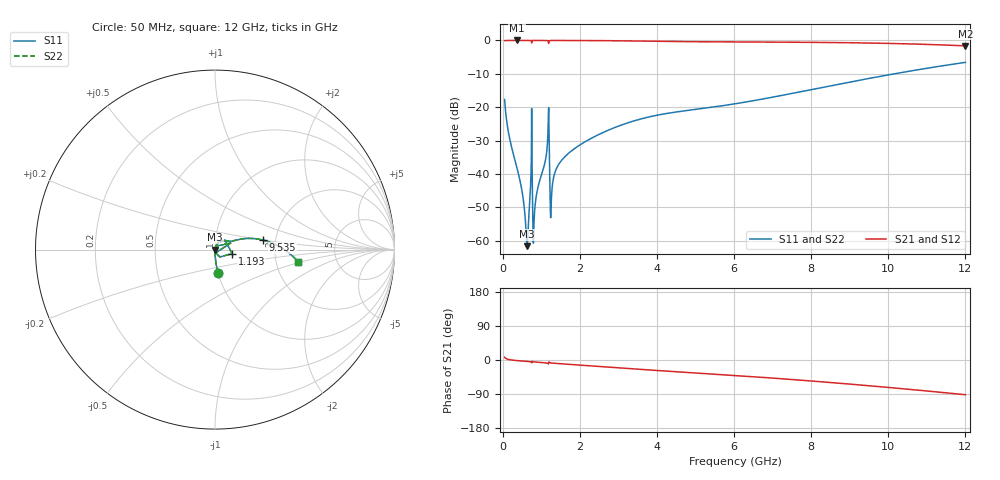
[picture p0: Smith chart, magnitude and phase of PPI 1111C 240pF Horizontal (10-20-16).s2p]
# MHz S MA R 50
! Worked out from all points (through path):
!   1601 points, 50 MHz to 12 GHz, reference 50 ohm
!   highest |S21| = -0.01 dB at 371.2 MHz (marker M1); lowest = -1.6 dB at 12 GHz (marker M2)
!   group delay of S21, straight-line fit = 20.7 ps
!   lowest |S11| = -61.7 dB at 632.6 MHz (marker M3), VSWR 1.00, Z = 50.1 - j0.0101 ohm
!   |S11| at or under -10 dB: start of sweep to 10.16 GHz
!   |S22| runs from -61.7 to -6.6 dB; largest |S21 - S12| = 0
!   S11 on the Smith chart (normalised r, x): 50 MHz: 1.00, -0.26; 1.193 GHz: 1.21, -0.06; 9.535 GHz: 1.71, +0.20; 12 GHz: 2.67, -0.47
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50  0.1303 -82.7  0.9912 7.2  0.9912 7.2  0.1303 -82.7
184.4375  0.03309 -88.4  0.999 0.8  0.999 0.8  0.03309 -88.4
371.1562  0.01226 -88.6  0.9993 -1.5  0.9993 -1.5  0.01226 -88.6
632.5625  0.0008261 -7.0  0.9991 -3.8  0.9991 -3.8  0.0008261 -7.0
669.9062  0.001914 58.4  0.9991 -4.1  0.9991 -4.1  0.001914 58.4
714.7188  0.005271 73.5  0.9989 -4.6  0.9989 -4.6  0.005271 73.5
796.875  0.000917 16.4  0.9991 -4.8  0.9991 -4.8  0.000917 16.4
834.2188  0.003074 68.3  0.9991 -5.2  0.9991 -5.2  0.003074 68.3
908.9062  0.00609 75.2  0.999 -5.8  0.999 -5.8  0.00609 75.2
1095.625  0.01474 76.9  0.9984 -7.4  0.9984 -7.4  0.01474 76.9
1140.438  0.02106 75.3  0.9973 -8.0  0.9973 -8.0  0.02106 75.3
1192.719  0.09836 -13.3  0.9022 -6.5  0.9022 -6.5  0.09836 -13.3
1282.344  0.006215 68.3  0.9984 -8.0  0.9984 -8.0  0.006215 68.3
1357.031  0.01062 74.0  0.9985 -8.7  0.9985 -8.7  0.01062 74.0
1469.062  0.01437 74.6  0.9984 -9.6  0.9984 -9.6  0.01437 74.6
2044.156  0.02812 70.3  0.9966 -13.8  0.9966 -13.8  0.02812 70.3
4038.312  0.07645 41.0  0.9696 -27.9  0.9696 -27.9  0.07645 41.0
6025  0.1124 25.8  0.9496 -40.8  0.9496 -40.8  0.1124 25.8
8019.156  0.1839 19.6  0.9365 -55.5  0.9365 -55.5  0.1839 19.6
9535.312  0.272 11.3  0.9135 -68.2  0.9135 -68.2  0.272 11.3
10013.31  0.3055 8.0  0.9025 -72.5  0.9025 -72.5  0.3055 8.0
12000  0.4689 -8.4  0.8293 -91.6  0.8293 -91.6  0.4689 -8.4
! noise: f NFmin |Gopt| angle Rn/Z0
50  0.000368  0.8647  0.3797  0.0005838
1372  0.004203  0.7041  8.169  0.002773
2701  0.01334  0.8078  16.01  0.01418
4031  0.03199  0.8783  23.72  0.05446
5360  0.0456  0.8889  31.17  0.08287
6682  0.05215  0.8833  38.3  0.08653
8012  0.05717  0.8777  45.14  0.08622
9341  0.06237  0.8751  51.64  0.08743
1.067e+04  0.06823  0.8755  57.78  0.09087
1.2e+04  0.07495  0.8786  63.58  0.09667
